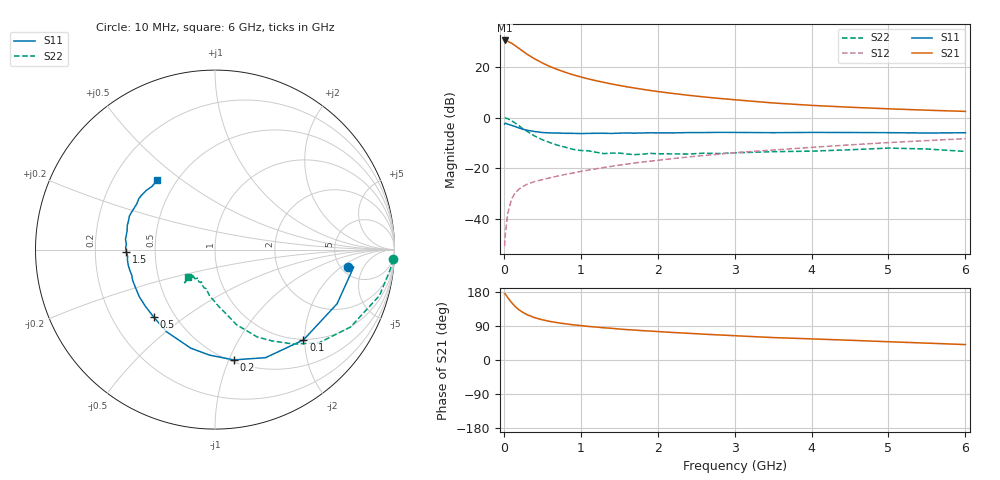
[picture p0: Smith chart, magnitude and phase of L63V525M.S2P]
!  INFINEON TECHNOLOGIES Small Signal Semiconductors
! BFR380L3 , Si-NPN RF-Transistor in TSLP-3-1
!  Vce=3.5 V,  Ic=25 mA
! Common Emitter S-Parameters:  07. March 2005
#  GHz  S  MA  R  50
! f  S11  S21  S12  S22
! GHz  Mag  Ang  Mag  Ang  Mag  Ang  Mag  Ang
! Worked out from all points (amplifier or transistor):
!   36 points, 10 MHz to 6 GHz, reference 50 ohm
!   highest |S21| = 30.5 dB at 10 MHz (marker M1)
!   |S21| within 3 dB of that: start of sweep to 190.4 MHz
!   unconditionally stable (mu >= 1): 1.943 GHz to 4.794 GHz
!   at 250 MHz: K = 0.37, MSG = 26.7 dB, |S12| = -27.2 dB
!   at 1.4 GHz: K = 0.95, MSG = 16.3 dB, |S12| = -19.2 dB
!   at 6 GHz: K = 0.97, MSG = 5.4 dB, |S12| = -8.3 dB
!   S11 on the Smith chart (normalised r, x): 10 MHz: 5.83, -2.52; 100 MHz: 0.99, -1.97; 200 MHz: 0.52, -1.04; 500 MHz: 0.38, -0.39; 1.5 GHz: 0.34, -0.01; 6 GHz: 0.39, +0.41
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0.01  0.7482 -7.3  33.41 175.0  0.0029 82.6  0.9953 -3.1
0.02  0.779 -7.1  33.4 173.9  0.0051 87.0  0.9829 -6.4
0.05  0.7442 -23.9  32.23 164.9  0.0126 80.1  0.9516 -15.6
0.1  0.7043 -45.6  29.46 151.7  0.0247 70.3  0.8699 -29.7
0.15  0.6648 -64.9  26.25 140.6  0.033 62.9  0.7785 -41.8
0.2  0.6233 -80.3  23.07 131.9  0.0392 58.9  0.6864 -50.1
0.25  0.5889 -92.9  20.36 125.4  0.0437 54.8  0.5999 -58.0
0.3  0.5654 -103.9  17.98 119.8  0.0484 53.7  0.5407 -64.2
0.4  0.5313 -120.5  14.49 111.7  0.0546 51.6  0.4345 -74.1
0.5  0.5082 -132.1  12.03 106.2  0.0597 52.2  0.3662 -79.8
0.6  0.4998 -141.2  10.2 101.7  0.0649 52.7  0.321 -85.7
0.7  0.4969 -148.0  8.885 98.4  0.0702 54.7  0.2852 -91.2
0.9  0.4898 -159.7  7.007 92.9  0.0807 56.7  0.2364 -100.3
1.1  0.4888 -166.8  5.816 88.6  0.0923 58.5  0.221 -106.1
1.5  0.4938 -178.6  4.329 81.7  0.1152 61.3  0.2001 -116.4
1.8  0.498 175.0  3.632 77.5  0.1329 62.3  0.1896 -122.1
2.2  0.5009 167.9  3.001 72.6  0.1556 63.1  0.1926 -125.7
2.8  0.5122 158.5  2.398 66.1  0.1901 63.8  0.1954 -132.9
3.5  0.5049 149.7  1.949 59.2  0.2297 62.3  0.2128 -132.6
4.5  0.5086 143.2  1.605 52.1  0.2902 61.2  0.2321 -132.7
5.5  0.4971 135.0  1.403 44.5  0.3522 58.0  0.2404 -132.6
6  0.5035 129.8  1.329 40.7  0.3847 56.0  0.2151 -134.3
